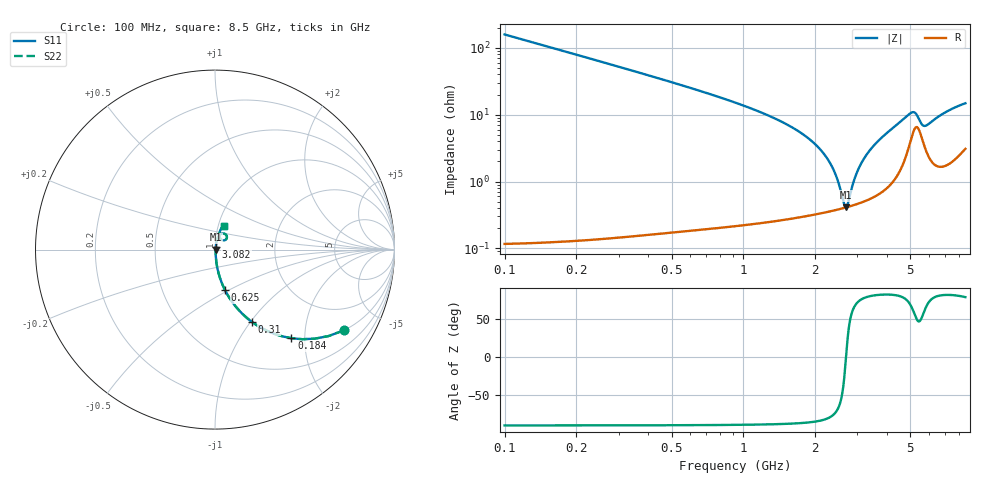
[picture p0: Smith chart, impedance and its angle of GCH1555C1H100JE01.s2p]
!Murata Part Number: GCH1555C1H100JE01
!These Parameters are Measured in Series Mode Connection
!Data Generated on Jun 19, 2026
!  o--ll--o
!Port1  Port2
!  o------o
!Operation Temp=25[degC], DC Bias Voltage=0[V]
!Freq. Start=100[MHz] Stop=9[GHz] 401[Steps]
# Hz S RI R 50
!Freq.(Hz) S11(Real) S11(Imag) S21(Real) S21(Imag) S12(Real) S12(Imag) S22(Real) S22(Imag)
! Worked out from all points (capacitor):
!   401 points, 100 MHz to 8.5 GHz, reference 50 ohm
!   read as one part in series: C = 10 pF near 142 MHz
!   lowest |Z| = 410 mohm at 2.683 GHz (marker M1)
!   series resonance near 2.689 GHz, so ESL is about 350 pH
!   S11 on the Smith chart (normalised r, x): 100 MHz: 1.00, -3.18; 184 MHz: 1.00, -1.72; 310 MHz: 1.00, -1.01; 625 MHz: 1.00, -0.48; 3.082 GHz: 1.01, +0.03; 8.5 GHz: 1.06, +0.29
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1e8  0.7162 -0.4505  0.2838 0.4505  0.2838 0.4505  0.7162 -0.4505
1.84e8  0.4256 -0.4937  0.5744 0.4937  0.5744 0.4937  0.4256 -0.4937
3.1e8  0.2047 -0.402  0.7953 0.402  0.7953 0.402  0.2047 -0.402
4.36e8  0.1131 -0.3144  0.8869 0.3144  0.8869 0.3144  0.1131 -0.3144
6.25e8  0.0563 -0.2267  0.9437 0.2267  0.9437 0.2267  0.0563 -0.2267
9.82e8  0.0214 -0.1371  0.9786 0.1371  0.9786 0.1371  0.0214 -0.1371
1.507e9  0.00789 -0.0719  0.9921 0.0719  0.9921 0.0719  0.00789 -0.0719
1.948e9  0.00466 -0.0388  0.9953 0.0388  0.9953 0.0388  0.00466 -0.0388
2.242e9  0.00396 -0.0218  0.996 0.0218  0.996 0.0218  0.00396 -0.0218
2.431e9  0.00387 -0.0121  0.9961 0.0121  0.9961 0.0121  0.00387 -0.0121
2.641e9  0.00401 -0.00218  0.996 0.00218  0.996 0.00218  0.00401 -0.00218
2.683e9  0.00407 -0.000289  0.9959 0.000289  0.9959 0.000289  0.00407 -0.000289
2.746e9  0.00417 0.0025  0.9958 -0.0025  0.9958 -0.0025  0.00417 0.0025
2.914e9  0.00453 0.00971  0.9955 -0.00971  0.9955 -0.00971  0.00453 0.00971
3.082e9  0.00503 0.0166  0.995 -0.0166  0.995 -0.0166  0.00503 0.0166
3.292e9  0.00583 0.025  0.9942 -0.025  0.9942 -0.025  0.00583 0.025
3.544e9  0.00711 0.0347  0.9929 -0.0347  0.9929 -0.0347  0.00711 0.0347
4.3e9  0.0148 0.0642  0.9852 -0.0642  0.9852 -0.0642  0.0148 0.0642
5.119e9  0.0574 0.0859  0.9426 -0.0859  0.9426 -0.0859  0.0574 0.0859
5.707e9  0.0369 0.0542  0.9631 -0.0542  0.9631 -0.0542  0.0369 0.0542
7.114e9  0.0287 0.1055  0.9713 -0.1055  0.9713 -0.1055  0.0287 0.1055
8.5e9  0.0488 0.1339  0.9512 -0.1339  0.9512 -0.1339  0.0488 0.1339
